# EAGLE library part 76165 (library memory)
MEMORY
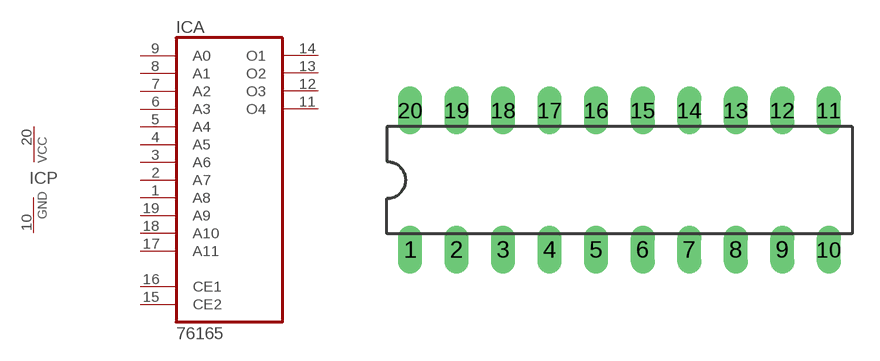
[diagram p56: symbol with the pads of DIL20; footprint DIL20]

Designator prefix IC; gates A=76165 P=PWRN

## 76165  [DIL20]
1  A:A8  in
2  A:A7  in
3  A:A6  in
4  A:A5  in
5  A:A4  in
6  A:A3  in
7  A:A2  in
8  A:A1  in
9  A:A0  in
10  P:GND  pwr
11  A:O4  hiz
12  A:O3  hiz
13  A:O2  hiz
14  A:O1  hiz
15  A:CE2  in
16  A:CE1  in
17  A:A11  in
18  A:A10  in
19  A:A9  in
20  P:VCC  pwr

## Footprint DIL20 (pad centres in mm)
Dual In Line Package
drill 0.813 long: 1 -11.43,-3.81; 2 -8.89,-3.81; 3 -6.35,-3.81; 4 -3.81,-3.81; 5 -1.27,-3.81; 6 1.27,-3.81; 7 3.81,-3.81; 8 6.35,-3.81; 9 8.89,-3.81; 10 11.43,-3.81; 11 11.43,3.81; 12 8.89,3.81; 13 6.35,3.81; 14 3.81,3.81; 15 1.27,3.81; 16 -1.27,3.81; 17 -3.81,3.81; 18 -6.35,3.81; 19 -8.89,3.81; 20 -11.43,3.81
